| IBIS file was generated by Viper version: 2022.03.25
[IBIS Ver]   4.2
[Comment Char]   |_char
[File Name]   n5xx_150mhz_100hlqfp_14x14_p02g.ibs
[File Rev]   1.0
[Date]   Mon Apr  4 13:26:25 2022
[Source]   NXP Viper 2022.03.25
[Notes]
[Disclaimer] IMPORTANT NOTICE
  This information is provided on an AS IS basis and without warranty.
  IN NO EVENT SHALL NXP BE LIABLE FOR INCIDENTAL OR CONSEQUENTIAL
  DAMAGES ARISING FROM USE OF THIS INFORMATION. THIS DISCLAIMER OF
  WARRANTY EXTENDS TO THE USER OF THE INFORMATION, AND TO THEIR CUSTOMERS
  OR USERS OF PRODUCTS  AND IS IN LIEU OF ALL WARRANTIES WHETHER EXPRESS,
  IMPLIED, OR STATUTORY, INCLUDING IMPLIED WARRANTIES OF MERCHANTABILITY
  OR FITNESS FOR PARTICULAR PURPOSE.
  NXP does not represent or warrant that the information furnished
  hereunder is free of infringement of any third party patents,
  copyrights, trade secrets, or other intellectual property rights.
  NXP does not represent or warrant that the information is free of
  defect, or that it meets any particular standard, requirements or need
  of the user of the infomation or their customers.
  NXP reserves the right to change the information in this file
  without notice.
   http://www.nxp.com
[Copyright]   (C) Copyright NXP 2004 - 2022, All Rights Reserved.
|   MCXN_100HLQFP_14x14_N5XX
[Component]   MCXN_100HLQFP_14x14_N5XX
[Manufacturer]   NXP
[Package]
| variable   typ   min   max
R_pkg   0.21486   0.10539   0.25442
L_pkg   4.761e-09   3.775e-09   5.668e-09
C_pkg   2.964e-13   2.489e-13   5.413e-13
[Pin] signal_name   model_name   R_pin   L_pin   C_pin
1   P1_8   a_ip_io_3v_3p3v   0.23595   5.586e-09 3.175e-13
2   P1_9   a_ip_io_3v_3p3v   0.22855   5.218e-09 3.123e-13
3   P1_10   a_ip_io_3v_3p3v   0.22439   5.125e-09 3.051e-13
4   P1_11   a_ip_io_3v_3p3v   0.22075   5.055e-09 3.000e-13
5   P1_12   a_ip_io_3v_3p3v   0.21788   4.926e-09 2.960e-13
6   P1_13   a_ip_io_3v_3p3v   0.21931   4.810e-09 2.924e-13
7   P1_14   a_ip_io_3v_3p3v   0.22439   4.733e-09 2.885e-13
8   P1_15   a_ip_io_3v_3p3v   0.23557   4.644e-09 2.860e-13
9   RESET_B   a_ip_io_3v_3p3v   0.22555   4.683e-09 2.707e-13
10   P1_30   a_ip_io_3v_3p3v   0.22909   4.673e-09 2.742e-13
11   P1_31   a_ip_io_3v_3p3v   0.23946   4.569e-09 2.743e-13
12   VDD_CORE   POWER   NA   NA   NA
13   VDD   POWER   NA   NA   NA
14   P2_0   a_ip_io_3v_1p8v   0.24948   4.735e-09 2.691e-13
15   P2_1   a_ip_io_3v_1p8v   0.2334   4.692e-09 2.722e-13
16   P2_2   a_ip_io_3v_1p8v   0.22783   4.693e-09 2.768e-13
17   P2_3   a_ip_io_3v_1p8v   0.22749   4.686e-09 2.826e-13
18   P2_4   a_ip_io_3v_1p8v   0.23132   4.759e-09 2.882e-13
19   P2_5   a_ip_io_3v_1p8v   0.24111   4.743e-09 2.946e-13
20   P2_6   a_ip_io_3v_1p8v   0.23817   4.937e-09 2.970e-13
21   P2_7   a_ip_io_3v_1p8v   0.24198   5.039e-09 3.020e-13
22   P4_0   a_ip_io_3v_3p3v   0.13479   4.564e-09 3.404e-13
23   P4_1   a_ip_io_3v_3p3v   0.13754   4.691e-09 3.561e-13
24   P4_2   a_ip_io_3v_3p3v   0.22936   5.299e-09 3.159e-13
25   P4_3   a_ip_io_3v_3p3v   0.23346   5.342e-09 3.178e-13
26   P4_4   a_ip_io_3v_3p3v   0.14373   4.982e-09 3.658e-13
27   P4_5   a_ip_io_3v_3p3v   0.14167   4.773e-09 3.660e-13
28   P4_6   a_ip_io_3v_3p3v   0.14515   4.630e-09 3.575e-13
29   P4_7   a_ip_io_3v_3p3v   0.10939   4.083e-09 3.972e-13
30   VDD_ANA   POWER   NA   NA   NA
31   VREFH   POWER   0.1252   4.073e-09 3.338e-13
32   VREFL   GND   0.20889   4.453e-09 2.810e-13
33   VSS_P4   GND   NA   NA   NA
34   VDD_P4   POWER   NA   NA   NA
35   P4_12   a_ip_io_3v_3p3v   0.21118   4.235e-09 2.656e-13
36   P4_13   a_ip_io_3v_3p3v   0.12896   3.995e-09 3.004e-13
37   P4_15   a_ip_io_3v_3p3v   0.21951   4.675e-09 2.489e-13
38   P4_16   a_ip_io_3v_3p3v   0.22761   4.784e-09 2.541e-13
39   P4_17   a_ip_io_3v_3p3v   0.13827   4.349e-09 2.908e-13
40   USB1_DP   NC   0.22533   4.468e-09 2.614e-13
41   USB1_DM   NC   0.21115   4.430e-09 2.603e-13
42   USB1_VBUS   POWER   0.20652   4.360e-09 2.628e-13
43   VSS   GND   NA   NA   NA
44   VDD_USB   POWER   NA   NA   NA
45   USB0_DM   NC   0.20763   4.303e-09 2.847e-13
46   USB0_DP   NC   0.21496   4.369e-09 2.938e-13
47   VDD_BAT   POWER   NA   NA   NA
48   P5_0   a_ip_io_3v_1p8v   0.22141   4.821e-09 3.018e-13
49   P5_1   a_ip_io_3v_1p8v   0.22331   4.979e-09 3.126e-13
50   P5_2   a_ip_io_3v_1p8v   0.23182   5.322e-09 3.185e-13
51   P5_3   a_ip_io_3v_1p8v   0.23252   5.145e-09 3.137e-13
52   VSS_DCDC   GND   NA   NA   NA
53   DCDC_LX   NC   0.10539   3.775e-09 5.413e-13
54   VDD_DCDC   POWER   NA   NA   NA
55   VDD_SYS   POWER   NA   NA   NA
56   P3_21   a_ip_io_3v_1p8v   0.25442   4.845e-09 3.109e-13
57   P3_20   a_ip_io_3v_1p8v   0.24759   4.705e-09 3.014e-13
58   VDD_CORE   POWER   NA   NA   NA
59   VDD_P3   POWER   NA   NA   NA
60   P3_17   a_ip_io_3v_1p8v   0.25062   4.783e-09 2.894e-13
61   P3_16   a_ip_io_3v_1p8v   0.24553   4.817e-09 2.841e-13
62   P3_15   a_ip_io_3v_1p8v   0.24794   4.958e-09 2.738e-13
63   P3_14   a_ip_io_3v_1p8v   0.25028   5.033e-09 2.708e-13
64   P3_13   a_ip_io_3v_1p8v   0.24346   4.922e-09 2.683e-13
65   P3_12   a_ip_io_3v_1p8v   0.23784   4.641e-09 2.718e-13
66   VDD_P3   POWER   NA   NA   NA
67   P3_11   a_ip_io_3v_1p8v   0.22732   4.472e-09 2.824e-13
68   P3_10   a_ip_io_3v_1p8v   0.22234   4.632e-09 2.841e-13
69   P3_9   a_ip_io_3v_1p8v   0.22368   4.771e-09 2.890e-13
70   P3_8   a_ip_io_3v_1p8v   0.22608   4.832e-09 2.967e-13
71   P3_7   a_ip_io_3v_1p8v   0.2327   4.958e-09 3.043e-13
72   P3_6   a_ip_io_3v_1p8v   0.24711   4.958e-09 3.154e-13
73   VDD_P3   POWER   NA   NA   NA
74   P3_1   a_ip_io_3v_1p8v   0.23381   5.181e-09 3.132e-13
75   P3_0   a_ip_io_3v_1p8v   0.24   5.373e-09 3.210e-13
76   P0_0   a_ip_io_3v_3p3v   0.24486   5.668e-09 3.238e-13
77   P0_1   a_ip_io_3v_3p3v   0.23554   5.440e-09 3.190e-13
78   P0_2   a_ip_io_3v_3p3v   0.22278   5.017e-09 3.080e-13
79   P0_3   a_ip_io_3v_3p3v   0.2128   4.789e-09 2.989e-13
80   P0_4   a_ip_io_3v_3p3v   0.20522   4.615e-09 2.903e-13
81   P0_5   a_ip_io_3v_3p3v   0.20257   4.533e-09 2.820e-13
82   P0_6   a_ip_io_3v_3p3v   0.20296   4.534e-09 2.696e-13
83   VDD   POWER   NA   NA   NA
84   P0_16   a_ip_io_3v_3p3v   0.22174   4.566e-09 2.717e-13
85   P0_17   a_ip_io_3v_3p3v   0.21775   4.594e-09 2.689e-13
86   P0_18   a_ip_io_3v_3p3v   0.21764   4.660e-09 2.624e-13
87   P0_19   a_ip_io_3v_3p3v   0.22279   4.781e-09 2.542e-13
88   P0_20   a_ip_io_3v_3p3v   0.22753   4.864e-09 2.516e-13
89   P0_21   a_ip_io_3v_3p3v   0.22243   4.836e-09 2.516e-13
90   P0_22   a_ip_io_3v_3p3v   0.2166   4.634e-09 2.593e-13
91   P0_23   a_ip_io_3v_3p3v   0.21934   4.486e-09 2.629e-13
92   P1_0   a_ip_io_3v_3p3v   0.20558   4.496e-09 2.606e-13
93   P1_1   a_ip_io_3v_3p3v   0.20276   4.476e-09 2.696e-13
94   P1_2   a_ip_io_3v_3p3v   0.20461   4.526e-09 2.751e-13
95   P1_3   a_ip_io_3v_3p3v   0.20833   4.488e-09 2.834e-13
96   VDD   POWER   NA   NA   NA
97   P1_4   a_ip_io_3v_3p3v   0.21547   4.670e-09 2.938e-13
98   P1_5   a_ip_io_3v_3p3v   0.21832   5.029e-09 2.996e-13
99   P1_6   a_ip_io_3v_3p3v   0.22077   5.126e-09 3.101e-13
100   P1_7   a_ip_io_3v_3p3v   0.2278   5.250e-09 3.150e-13
101   VSS   GND   NA   NA   NA
[Pin Mapping]   pulldown_ref   pullup_ref
1   NC   NC
2   NC   NC
3   NC   NC
4   NC   NC
5   NC   NC
6   NC   NC
7   NC   NC
8   NC   NC
9   NC   NC
10   NC   NC
11   NC   NC
12   NC   VDD_CORE
13   NC   VDD
14   NC   NC
15   NC   NC
16   NC   NC
17   NC   NC
18   NC   NC
19   NC   NC
20   NC   NC
21   NC   NC
22   NC   NC
23   NC   NC
24   NC   NC
25   NC   NC
26   NC   NC
27   NC   NC
28   NC   NC
29   NC   NC
30   NC   VDD_ANA
31   NC   VREFH
32   VREFL   NC
33   VSS_P4   NC
34   NC   VDD_P4
35   NC   NC
36   NC   NC
37   NC   NC
38   NC   NC
39   NC   NC
40   NC   NC
41   NC   NC
42   NC   USB1_VBUS
43   VSS   NC
44   NC   VDD_USB
45   NC   NC
46   NC   NC
47   NC   VDD_BAT
48   NC   NC
49   NC   NC
50   NC   NC
51   NC   NC
52   VSS_DCDC   NC
53   NC   NC
54   NC   VDD_DCDC
55   NC   VDD_SYS
56   NC   NC
57   NC   NC
58   NC   VDD_CORE
59   NC   VDD_P3
60   NC   NC
61   NC   NC
62   NC   NC
63   NC   NC
64   NC   NC
65   NC   NC
66   NC   VDD_P3
67   NC   NC
68   NC   NC
69   NC   NC
70   NC   NC
71   NC   NC
72   NC   NC
73   NC   VDD_P3
74   NC   NC
75   NC   NC
76   NC   NC
77   NC   NC
78   NC   NC
79   NC   NC
80   NC   NC
81   NC   NC
82   NC   NC
83   NC   VDD
84   NC   NC
85   NC   NC
86   NC   NC
87   NC   NC
88   NC   NC
89   NC   NC
90   NC   NC
91   NC   NC
92   NC   NC
93   NC   NC
94   NC   NC
95   NC   NC
96   NC   VDD
97   NC   NC
98   NC   NC
99   NC   NC
100   NC   NC
101   VSS   NC
|*   Model Selector   *
[Model Selector] a_ip_io_3v_1p8v
p_io_25mhz_ds0_sr0_1p8v_mio   dse=0 sre=0 25mhz
p_io_25mhz_ds0_sr1_1p8v_mio   dse=0 sre=1 25mhz
p_io_25mhz_ds1_sr0_1p8v_mio   dse=1 sre=0 25mhz
p_io_25mhz_ds1_sr1_1p8v_mio   dse=1 sre=1 25mhz
p_io_25mhz_r40_ds0_sr0_1p8v_mio   dse=0 sre=0 25mhz_r40
p_io_25mhz_r40_ds0_sr1_1p8v_mio   dse=0 sre=1 25mhz_r40
p_io_25mhz_r40_ds1_sr0_1p8v_mio   dse=1 sre=0 25mhz_r40
p_io_25mhz_r40_ds1_sr1_1p8v_mio   dse=1 sre=1 25mhz_r40
p_io_50mhz_ds0_sr0_1p8v_mio   dse=0 sre=0 50mhz
p_io_50mhz_ds0_sr1_1p8v_mio   dse=0 sre=1 50mhz
p_io_50mhz_ds1_sr0_1p8v_mio   dse=1 sre=0 50mhz
p_io_50mhz_ds1_sr1_1p8v_mio   dse=1 sre=1 50mhz
p_io_25mhz_cap_ds0_sr0_1p8v_mio   dse=0 sre=0 25mhz_cap
p_io_25mhz_cap_ds0_sr1_1p8v_mio   dse=0 sre=1 25mhz_cap
p_io_25mhz_cap_ds1_sr0_1p8v_mio   dse=1 sre=0 25mhz_cap
p_io_25mhz_cap_ds1_sr1_1p8v_mio   dse=1 sre=1 25mhz_cap
p_io_25mhz_2mux_ds0_sr0_1p8v_mio   dse=0 sre=0 25mhz_2mux
p_io_25mhz_2mux_ds0_sr1_1p8v_mio   dse=0 sre=1 25mhz_2mux
p_io_25mhz_2mux_ds1_sr0_1p8v_mio   dse=1 sre=0 25mhz_2mux
p_io_25mhz_2mux_ds1_sr1_1p8v_mio   dse=1 sre=1 25mhz_2mux
p_io_100mhz_ds0_sr0_1p8v_mio   dse=0 sre=0 100mhz
p_io_100mhz_ds0_sr1_1p8v_mio   dse=0 sre=1 100mhz
p_io_100mhz_ds1_sr0_1p8v_mio   dse=1 sre=0 100mhz
p_io_100mhz_ds1_sr1_1p8v_mio   dse=1 sre=1 100mhz
p_io_100mhz_weftd_ds0_sr0_1p8v_mio   dse=0 sre=0 100mhz
p_io_100mhz_weftd_ds0_sr1_1p8v_mio   dse=0 sre=1 100mhz
p_io_100mhz_weftd_ds1_sr0_1p8v_mio   dse=1 sre=0 100mhz
p_io_100mhz_weftd_ds1_sr1_1p8v_mio   dse=1 sre=1 100mhz
p_io_i2c_ds00_ds10_sr0_1p8v_mio   dse0=0 dse1=0 sre=0 i2c
p_io_i2c_ds00_ds10_sr1_1p8v_mio   dse0=0 dse1=0 sre=1 i2c
p_io_i2c_ds00_ds11_sr0_1p8v_mio   dse0=0 dse1=1 sre=0 i2c
p_io_i2c_ds00_ds11_sr1_1p8v_mio   dse0=0 dse1=1 sre=1 i2c
p_io_i2c_ds01_ds10_sr0_1p8v_mio   dse0=1 dse1=0 sre=0 i2c
p_io_i2c_ds01_ds10_sr1_1p8v_mio   dse0=1 dse1=0 sre=1 i2c
p_io_i2c_ds01_ds11_sr0_1p8v_mio   dse0=1 dse1=1 sre=0 i2c
p_io_i2c_ds01_ds11_sr1_1p8v_mio   dse0=1 dse1=1 sre=1 i2c
p_io_i2c_i2c1_1p8v_mio   ipp_i2c_lv=1 i2c
p_io_i2cfmp_ds00_ds10_sr0_1p8v_mio   dse0=0 dse1=0 sre=0 i2cfmp
p_io_i2cfmp_ds00_ds10_sr1_1p8v_mio   dse0=0 dse1=0 sre=1 i2cfmp
p_io_i2cfmp_ds00_ds11_sr0_1p8v_mio   dse0=0 dse1=1 sre=0 i2cfmp
p_io_i2cfmp_ds00_ds11_sr1_1p8v_mio   dse0=0 dse1=1 sre=1 i2cfmp
p_io_i2cfmp_ds01_ds10_sr0_1p8v_mio   dse0=1 dse1=0 sre=0 i2cfmp
p_io_i2cfmp_ds01_ds10_sr1_1p8v_mio   dse0=1 dse1=0 sre=1 i2cfmp
p_io_i2cfmp_ds01_ds11_sr0_1p8v_mio   dse0=1 dse1=1 sre=0 i2cfmp
p_io_i2cfmp_ds01_ds11_sr1_1p8v_mio   dse0=1 dse1=1 sre=1 i2cfmp
p_io_i2cfmp_i2c1_1p8v_mio   ipp_i2c_lv=1 i2cfmp
p_io_rst_1p8v_mio   rst
p_io_rst_rx1p8v_1p8v_mio   rst
p_io_aon_1p8v_mio   rst
[Model Selector] a_ip_io_3v_3p3v
p_io_25mhz_ds0_sr0_3p3v_mio   dse=0 sre=0 25mhz
p_io_25mhz_ds0_sr1_3p3v_mio   dse=0 sre=1 25mhz
p_io_25mhz_ds1_sr0_3p3v_mio   dse=1 sre=0 25mhz
p_io_25mhz_ds1_sr1_3p3v_mio   dse=1 sre=1 25mhz
p_io_25mhz_r40_ds0_sr0_3p3v_mio   dse=0 sre=0 25mhz_r40
p_io_25mhz_r40_ds0_sr1_3p3v_mio   dse=0 sre=1 25mhz_r40
p_io_25mhz_r40_ds1_sr0_3p3v_mio   dse=1 sre=0 25mhz_r40
p_io_25mhz_r40_ds1_sr1_3p3v_mio   dse=1 sre=1 25mhz_r40
p_io_50mhz_ds0_sr0_3p3v_mio   dse=0 sre=0 50mhz
p_io_50mhz_ds0_sr1_3p3v_mio   dse=0 sre=1 50mhz
p_io_50mhz_ds1_sr0_3p3v_mio   dse=1 sre=0 50mhz
p_io_50mhz_ds1_sr1_3p3v_mio   dse=1 sre=1 50mhz
p_io_25mhz_cap_ds0_sr0_3p3v_mio   dse=0 sre=0 25mhz_cap
p_io_25mhz_cap_ds0_sr1_3p3v_mio   dse=0 sre=1 25mhz_cap
p_io_25mhz_cap_ds1_sr0_3p3v_mio   dse=1 sre=0 25mhz_cap
p_io_25mhz_cap_ds1_sr1_3p3v_mio   dse=1 sre=1 25mhz_cap
p_io_25mhz_2mux_ds0_sr0_3p3v_mio   dse=0 sre=0 25mhz_2mux
p_io_25mhz_2mux_ds0_sr1_3p3v_mio   dse=0 sre=1 25mhz_2mux
p_io_25mhz_2mux_ds1_sr0_3p3v_mio   dse=1 sre=0 25mhz_2mux
p_io_25mhz_2mux_ds1_sr1_3p3v_mio   dse=1 sre=1 25mhz_2mux
p_io_100mhz_ds0_sr0_3p3v_mio   dse=0 sre=0 100mhz
p_io_100mhz_ds0_sr1_3p3v_mio   dse=0 sre=1 100mhz
p_io_100mhz_ds1_sr0_3p3v_mio   dse=1 sre=0 100mhz
p_io_100mhz_ds1_sr1_3p3v_mio   dse=1 sre=1 100mhz
p_io_100mhz_weftd_ds0_sr0_3p3v_mio   dse=0 sre=0 100mhz
p_io_100mhz_weftd_ds0_sr1_3p3v_mio   dse=0 sre=1 100mhz
p_io_100mhz_weftd_ds1_sr0_3p3v_mio   dse=1 sre=0 100mhz
p_io_100mhz_weftd_ds1_sr1_3p3v_mio   dse=1 sre=1 100mhz
p_io_i2c_ds00_ds10_sr0_3p3v_mio   dse0=0 dse1=0 sre=0 i2c
p_io_i2c_ds00_ds10_sr1_3p3v_mio   dse0=0 dse1=0 sre=1 i2c
p_io_i2c_ds00_ds11_sr0_3p3v_mio   dse0=0 dse1=1 sre=0 i2c
p_io_i2c_ds00_ds11_sr1_3p3v_mio   dse0=0 dse1=1 sre=1 i2c
p_io_i2c_ds01_ds10_sr0_3p3v_mio   dse0=1 dse1=0 sre=0 i2c
p_io_i2c_ds01_ds10_sr1_3p3v_mio   dse0=1 dse1=0 sre=1 i2c
p_io_i2c_ds01_ds11_sr0_3p3v_mio   dse0=1 dse1=1 sre=0 i2c
p_io_i2c_ds01_ds11_sr1_3p3v_mio   dse0=1 dse1=1 sre=1 i2c
p_io_i2c_i2c1_3p3v_mio   ipp_i2c_lv=1 i2c
p_io_i2cfmp_ds00_ds10_sr0_3p3v_mio   dse0=0 dse1=0 sre=0 i2cfmp
p_io_i2cfmp_ds00_ds10_sr1_3p3v_mio   dse0=0 dse1=0 sre=1 i2cfmp
p_io_i2cfmp_ds00_ds11_sr0_3p3v_mio   dse0=0 dse1=1 sre=0 i2cfmp
p_io_i2cfmp_ds00_ds11_sr1_3p3v_mio   dse0=0 dse1=1 sre=1 i2cfmp
p_io_i2cfmp_ds01_ds10_sr0_3p3v_mio   dse0=1 dse1=0 sre=0 i2cfmp
p_io_i2cfmp_ds01_ds10_sr1_3p3v_mio   dse0=1 dse1=0 sre=1 i2cfmp
p_io_i2cfmp_ds01_ds11_sr0_3p3v_mio   dse0=1 dse1=1 sre=0 i2cfmp
p_io_i2cfmp_ds01_ds11_sr1_3p3v_mio   dse0=1 dse1=1 sre=1 i2cfmp
p_io_i2cfmp_i2c1_3p3v_mio   ipp_i2c_lv=1 i2cfmp
p_io_rst_3p3v_mio   rst
p_io_rst_rx1p8v_3p3v_mio   rst
p_io_aon_3p3v_mio   rst
| End [Component] MCXN_100HLQFP_14x14_N5XX
| Models and submodels in the file (98): p_io_100mhz_ds0_sr0_1p8v_mio (I/O), p_io_100mhz_ds0_sr0_3p3v_mio (I/O), p_io_100mhz_ds0_sr1_1p8v_mio (I/O), p_io_100mhz_ds0_sr1_3p3v_mio (I/O), p_io_100mhz_ds1_sr0_1p8v_mio (I/O), p_io_100mhz_ds1_sr0_3p3v_mio (I/O), p_io_100mhz_ds1_sr1_1p8v_mio (I/O), p_io_100mhz_ds1_sr1_3p3v_mio (I/O), p_io_100mhz_weftd_ds0_sr0_1p8v_mio (I/O), p_io_100mhz_weftd_ds0_sr0_3p3v_mio (I/O), p_io_100mhz_weftd_ds0_sr1_1p8v_mio (I/O), p_io_100mhz_weftd_ds0_sr1_3p3v_mio (I/O), p_io_100mhz_weftd_ds1_sr0_1p8v_mio (I/O), p_io_100mhz_weftd_ds1_sr0_3p3v_mio (I/O), p_io_100mhz_weftd_ds1_sr1_1p8v_mio (I/O), p_io_100mhz_weftd_ds1_sr1_3p3v_mio (I/O), p_io_25mhz_2mux_ds0_sr0_1p8v_mio (I/O), p_io_25mhz_2mux_ds0_sr0_3p3v_mio (I/O), p_io_25mhz_2mux_ds0_sr1_1p8v_mio (I/O), p_io_25mhz_2mux_ds0_sr1_3p3v_mio (I/O), p_io_25mhz_2mux_ds1_sr0_1p8v_mio (I/O), p_io_25mhz_2mux_ds1_sr0_3p3v_mio (I/O), p_io_25mhz_2mux_ds1_sr1_1p8v_mio (I/O), p_io_25mhz_2mux_ds1_sr1_3p3v_mio (I/O), p_io_25mhz_cap_ds0_sr0_1p8v_mio (I/O), p_io_25mhz_cap_ds0_sr0_3p3v_mio (I/O), p_io_25mhz_cap_ds0_sr1_1p8v_mio (I/O), p_io_25mhz_cap_ds0_sr1_3p3v_mio (I/O), p_io_25mhz_cap_ds1_sr0_1p8v_mio (I/O), p_io_25mhz_cap_ds1_sr0_3p3v_mio (I/O), p_io_25mhz_cap_ds1_sr1_1p8v_mio (I/O), p_io_25mhz_cap_ds1_sr1_3p3v_mio (I/O), p_io_25mhz_ds0_sr0_1p8v_mio (I/O), p_io_25mhz_ds0_sr0_3p3v_mio (I/O), p_io_25mhz_ds0_sr1_1p8v_mio (I/O), p_io_25mhz_ds0_sr1_3p3v_mio (I/O), p_io_25mhz_ds1_sr0_1p8v_mio (I/O), p_io_25mhz_ds1_sr0_3p3v_mio (I/O), p_io_25mhz_ds1_sr1_1p8v_mio (I/O), p_io_25mhz_ds1_sr1_3p3v_mio (I/O), p_io_25mhz_r40_ds0_sr0_1p8v_mio (I/O), p_io_25mhz_r40_ds0_sr0_3p3v_mio (I/O), p_io_25mhz_r40_ds0_sr1_1p8v_mio (I/O), p_io_25mhz_r40_ds0_sr1_3p3v_mio (I/O), p_io_25mhz_r40_ds1_sr0_1p8v_mio (I/O), p_io_25mhz_r40_ds1_sr0_3p3v_mio (I/O), p_io_25mhz_r40_ds1_sr1_1p8v_mio (I/O), p_io_25mhz_r40_ds1_sr1_3p3v_mio (I/O), p_io_50mhz_ds0_sr0_1p8v_mio (I/O), p_io_50mhz_ds0_sr0_3p3v_mio (I/O), p_io_50mhz_ds0_sr1_1p8v_mio (I/O), p_io_50mhz_ds0_sr1_3p3v_mio (I/O), p_io_50mhz_ds1_sr0_1p8v_mio (I/O), p_io_50mhz_ds1_sr0_3p3v_mio (I/O), p_io_50mhz_ds1_sr1_1p8v_mio (I/O), p_io_50mhz_ds1_sr1_3p3v_mio (I/O), p_io_aon_1p8v_mio (I/O), p_io_aon_3p3v_mio (I/O), p_io_i2c_ds00_ds10_sr0_1p8v_mio (I/O), p_io_i2c_ds00_ds10_sr0_3p3v_mio (I/O), p_io_i2c_ds00_ds10_sr1_1p8v_mio (I/O), p_io_i2c_ds00_ds10_sr1_3p3v_mio (I/O), p_io_i2c_ds00_ds11_sr0_1p8v_mio (I/O), p_io_i2c_ds00_ds11_sr0_3p3v_mio (I/O), p_io_i2c_ds00_ds11_sr1_1p8v_mio (I/O), p_io_i2c_ds00_ds11_sr1_3p3v_mio (I/O), p_io_i2c_ds01_ds10_sr0_1p8v_mio (I/O), p_io_i2c_ds01_ds10_sr0_3p3v_mio (I/O), p_io_i2c_ds01_ds10_sr1_1p8v_mio (I/O), p_io_i2c_ds01_ds10_sr1_3p3v_mio (I/O), p_io_i2c_ds01_ds11_sr0_1p8v_mio (I/O), p_io_i2c_ds01_ds11_sr0_3p3v_mio (I/O), p_io_i2c_ds01_ds11_sr1_1p8v_mio (I/O), p_io_i2c_ds01_ds11_sr1_3p3v_mio (I/O), p_io_i2c_i2c1_1p8v_mio (I/O), p_io_i2c_i2c1_3p3v_mio (I/O), p_io_i2cfmp_ds00_ds10_sr0_1p8v_mio (I/O), p_io_i2cfmp_ds00_ds10_sr0_3p3v_mio (I/O), p_io_i2cfmp_ds00_ds10_sr1_1p8v_mio (I/O), p_io_i2cfmp_ds00_ds10_sr1_3p3v_mio (I/O)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
